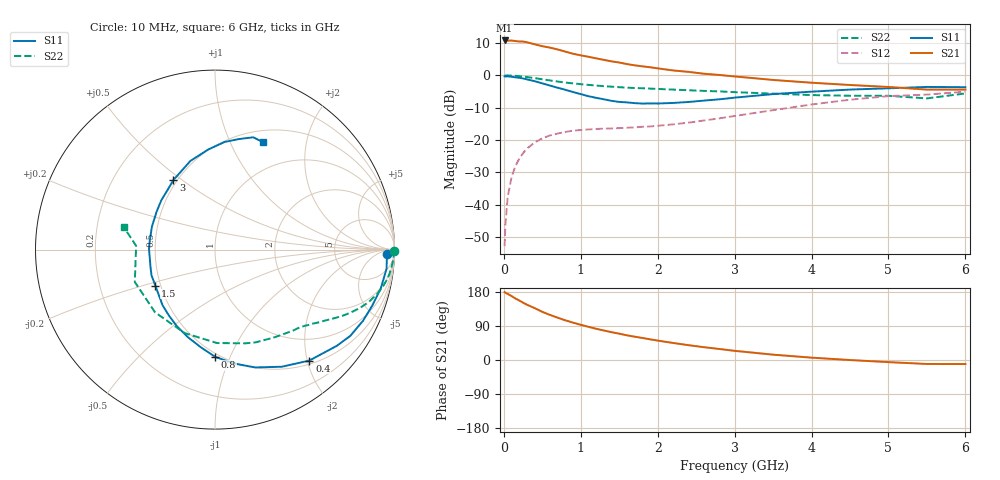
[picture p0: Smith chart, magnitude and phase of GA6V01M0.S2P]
! Infineon Technologies  Discrete & RF Semiconductors
! BF775
! Si NPN RF Bipolar Junction Transistor in SOT23
! VCE = 6 V  IC = 1 mA
! Common Emitter S-Parameters:  May  1996
# GHz  S  MA  R  50
!  f  S11  S21  S12  S22
! GHz  MAG  ANG  MAG  ANG  MAG  ANG  MAG  ANG
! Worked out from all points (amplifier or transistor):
!   36 points, 10 MHz to 6 GHz, reference 50 ohm
!   highest |S21| = 10.8 dB at 10 MHz (marker M1)
!   |S21| within 3 dB of that: start of sweep to 732.3 MHz
!   unconditionally stable (mu >= 1): 1.457 GHz to 3.686 GHz; 5.244 GHz to end of sweep
!   at 250 MHz: K = 0.20, MSG = 17.2 dB, |S12| = -24.0 dB
!   at 1.4 GHz: K = 0.97, MSG = 10.4 dB, |S12| = -16.4 dB
!   at 6 GHz: K = 1.00, MAG = 0.0 dB, |S12| = -5.1 dB
!   S11 on the Smith chart (normalised r, x): 10 MHz: 36, -22; 400 MHz: 0.56, -2.04; 800 MHz: 0.47, -0.88; 1.5 GHz: 0.47, -0.22; 3 GHz: 0.48, +0.46; 6 GHz: 0.64, +1.34
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0.01  0.9609 -1.4  3.45 179.2  0.0023 88.1  0.9999 -0.4
0.02  0.9586 -2.7  3.448 177.6  0.0049 88.2  0.9923 -1.0
0.05  0.9617 -6.3  3.424 174.4  0.0132 85.7  0.9961 -2.6
0.1  0.9488 -13.1  3.441 168.8  0.0266 81.7  0.9895 -5.3
0.15  0.9301 -19.6  3.379 162.4  0.0394 77.4  0.9809 -8.1
0.25  0.8941 -32.5  3.319 151.3  0.0628 70.0  0.9561 -12.7
0.3  0.8649 -38.3  3.238 145.9  0.0737 67.1  0.939 -15.0
0.4  0.8116 -49.6  3.011 137.0  0.0915 60.5  0.9052 -18.9
0.5  0.7513 -60.3  2.812 127.1  0.1063 55.3  0.8681 -22.1
0.6  0.6935 -71.2  2.673 118.9  0.118 50.4  0.8325 -25.0
0.8  0.5974 -89.9  2.318 104.7  0.1334 43.2  0.772 -29.5
0.9  0.5512 -98.0  2.149 98.5  0.1397 41.1  0.75 -31.2
1.1  0.476 -116.7  1.931 87.5  0.146 37.7  0.7108 -34.6
1.5  0.3881 -148.9  1.575 69.5  0.1529 36.1  0.6549 -40.5
1.9  0.3679 179.4  1.331 54.6  0.1622 38.6  0.6231 -46.9
2.2  0.374 160.1  1.188 45.0  0.1746 41.8  0.6014 -52.3
3  0.4516 120.9  0.96 24.2  0.2353 47.0  0.5494 -71.9
3.5  0.5127 105.5  0.847 14.1  0.2895 45.7  0.5207 -88.8
4.5  0.602 84.9  0.708 -0.1  0.4198 35.0  0.4834 -133.7
5  0.6297 77.9  0.66 -5.6  0.477 26.7  0.4819 -158.0
5.5  0.6611 71.2  0.601 -10.5  0.5035 17.1  0.4399 177.3
6  0.6553 65.7  0.602 -10.7  0.5581 12.2  0.5245 166.0
